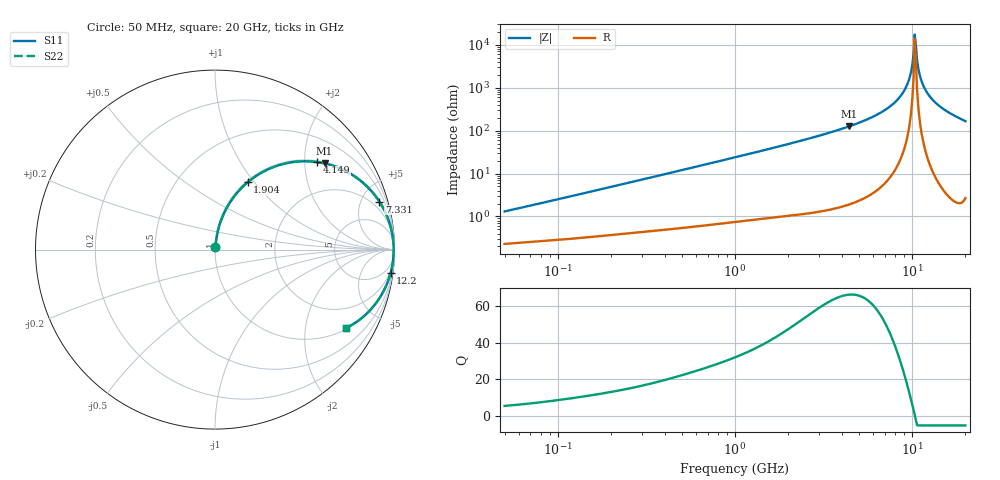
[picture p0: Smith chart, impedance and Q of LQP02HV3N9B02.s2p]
!Murata Part Number: LQP02HV3N9B02
!These Parameters are Measured in Series Mode Connection
!  o--[Z]--o
!Port1  Port2
!  o-------o
!Freq. Start=50[MHz] Stop=20[GHz], 401[Steps]
# Hz S RI R 50
!Freq.(Hz) S11(Real) S11(Imag) S21(Real) S21(Imag) S12(Real) S12(Imag) S22(Real) S22(Imag)
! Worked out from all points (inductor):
!   401 points, 50 MHz to 20 GHz, reference 50 ohm
!   read as one part in series: L = 4.06 nH near 51.52 MHz
!   highest Q = 66.1 at 4.406 GHz (marker M1), where L = 4.54 nH
!   self-resonance near 10.35 GHz
!   S11 on the Smith chart (normalised r, x): 50 MHz: 1.00, +0.03; 1.904 GHz: 1.02, +0.93; 4.149 GHz: 1.04, +2.31; 7.331 GHz: 1.14, +6.81; 12.2 GHz: 1, -15; 20 GHz: 1.05, -3.31
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5e7  0.00246 0.0129  0.9975 -0.0129  0.9975 -0.0129  0.00246 0.0129
1.364002e8  0.0043 0.0335  0.9957 -0.0335  0.9957 -0.0335  0.0043 0.0335
3.721004e8  0.0126 0.0882  0.9874 -0.0882  0.9874 -0.0882  0.0126 0.0882
1e9  0.0603 0.2229  0.9397 -0.2229  0.9397 -0.2229  0.0603 0.2229
1.904239e9  0.1818 0.375  0.8182 -0.375  0.8182 -0.375  0.1818 0.375
2.728004e9  0.3233 0.4589  0.6767 -0.4589  0.6767 -0.4589  0.3233 0.4589
4.149438e9  0.5703 0.4875  0.4297 -0.4875  0.4297 -0.4875  0.5703 0.4875
4.405649e9  0.6104 0.4802  0.3896 -0.4802  0.3896 -0.4802  0.6104 0.4802
5.856089e9  0.7969 0.3943  0.2031 -0.3943  0.2031 -0.3943  0.7969 0.3943
7.331367e9  0.916 0.2671  0.084 -0.2671  0.084 -0.2671  0.916 0.2671
7.442007e9  0.9223 0.257  0.0777 -0.257  0.0777 -0.257  0.9223 0.257
8.516016e9  0.9685 0.1591  0.0315 -0.1591  0.0315 -0.1591  0.9685 0.1591
9.316812e9  0.9871 0.0886  0.0129 -0.0886  0.0129 -0.0886  0.9871 0.0886
9.745021e9  0.9925 0.0523  0.00752 -0.0523  0.00752 -0.0523  0.9925 0.0523
1.019291e10  0.9951 0.0157  0.00486 -0.0157  0.00486 -0.0157  0.9951 0.0157
1.034674e10  0.9954 0.00343  0.00457 -0.00343  0.00457 -0.00343  0.9954 0.00343
1.066139e10  0.9951 -0.0211  0.00492 0.0211  0.00492 0.0211  0.9951 -0.0211
1.098561e10  0.9935 -0.0456  0.00648 0.0456  0.00648 0.0456  0.9935 -0.0456
1.131968e10  0.9907 -0.07  0.00925 0.07  0.00925 0.07  0.9907 -0.07
1.220001e10  0.9786 -0.13  0.0214 0.13  0.0214 0.13  0.9786 -0.13
1.482269e10  0.9137 -0.2742  0.0863 0.2742  0.0863 0.2742  0.9137 -0.2742
2e10  0.7298 -0.4361  0.2702 0.4361  0.2702 0.4361  0.7298 -0.4361
